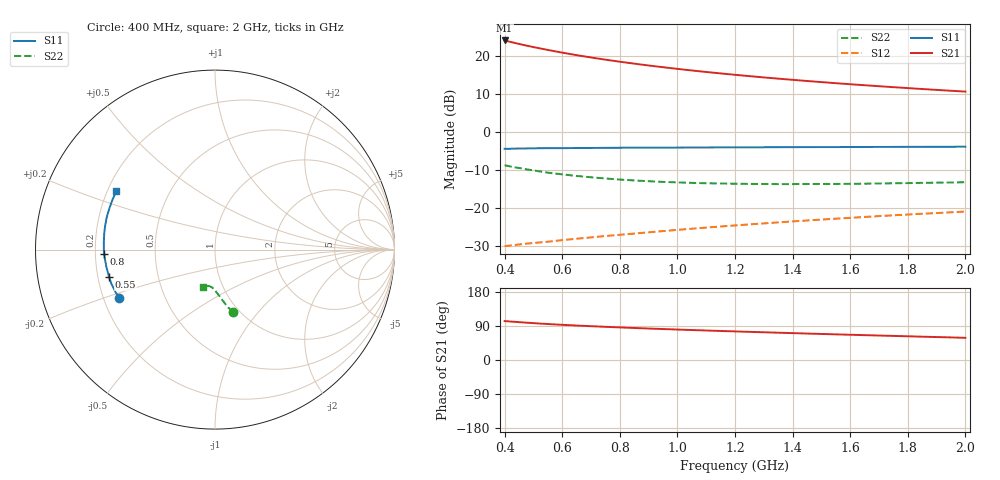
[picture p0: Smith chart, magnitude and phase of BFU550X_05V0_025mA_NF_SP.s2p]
! Filename:  P:\Prog\Test\Noise\ATS_data\Testdata_Net\BFU550X attenuator noise\BFU550X_APG2013_44_C05_05p0V_025mA_NF_CM01_D.sf
! Date/Time: Fri 26/Jul/2013 14:34:21
! BFU550X_APG2013_44_C05_05p0V_1to35mA_NF_CM01_Bias7_R.sf
! Noise Parameter Data File
! BFU550X_APG2013_44_C05_05p0V_1to35mA_NF_CM01
! Date/time: Mon Jul 22 09:12:23 2013
! VAR V_out= 5.001000
! VAR I_out= 25.005000
! VAR V_in= 0.825600
! VAR I_in= 0.279550
! Device data file deembeded for feedlines and parallel
! Original file: \BFU550X attenuator noise\BFU550X_APG2013_44_C05_05p0V_025mA_NF_CM01_R.sf
! Feed-files: PR005V01_100713_Feed1.s2p, PR005V01_100713_Feed2.s2p
! Parallel-file: PR005V01_100713_Par.s2p
# MHz S MA R 50
!  Freq-MHz  S11-mag  S11-arg  S21-mag  S21-arg  S12-mag  S12-arg  S22-mag  S22-arg
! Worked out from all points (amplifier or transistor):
!   37 points, 400 MHz to 2 GHz, reference 50 ohm
!   highest |S21| = 24.0 dB at 400 MHz (marker M1)
!   |S21| within 3 dB of that: start of sweep to 586.2 MHz
!   unconditionally stable (mu >= 1): 1.335 GHz to end of sweep
!   at 500 MHz: K = 0.69, MSG = 25.7 dB, |S12| = -29.2 dB
!   at 1.1 GHz: K = 0.96, MSG = 20.4 dB, |S12| = -25.1 dB
!   at 2 GHz: K = 1.05, MAG = 14.4 dB, |S12| = -20.9 dB
!   lowest NFmin = 1.11 dB at 480 MHz
!   S11 on the Smith chart (normalised r, x): 400 MHz: 0.26, -0.22; 550 MHz: 0.25, -0.12; 800 MHz: 0.24, -0.02; 2 GHz: 0.24, +0.26
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400  0.5995 -153.4  15.81 102.8  0.03158 47.9  0.3643 -74.0
420  0.5995 -155.2  15.13 101.6  0.03225 48.2  0.3512 -75.3
460  0.6038 -158.6  13.96 99.3  0.03356 48.5  0.3314 -77.2
480  0.6057 -160.2  13.43 98.3  0.03418 48.8  0.3198 -78.2
500  0.6076 -161.7  12.95 97.3  0.03476 49.0  0.312 -78.9
550  0.6103 -165.3  11.87 94.9  0.03612 49.9  0.2911 -80.9
600  0.6102 -168.1  10.95 92.9  0.0379 50.7  0.2767 -82.6
650  0.613 -170.8  10.14 91.0  0.03954 51.4  0.2635 -84.1
700  0.6138 -173.2  9.455 89.2  0.04115 52.2  0.253 -85.6
750  0.6161 -175.5  8.849 87.6  0.04293 52.9  0.2441 -86.9
800  0.6183 -177.6  8.321 86.0  0.04455 53.5  0.2364 -88.3
850  0.6193 -179.7  7.848 84.5  0.04621 54.1  0.23 -89.5
900  0.6194 178.5  7.421 83.1  0.04799 54.8  0.2248 -90.6
950  0.6207 176.7  7.045 81.7  0.04981 55.3  0.2202 -91.6
1050  0.622 173.4  6.387 79.1  0.05352 56.2  0.2137 -93.6
1100  0.6235 171.9  6.101 77.8  0.05536 56.6  0.2113 -94.5
1200  0.6253 168.9  5.602 75.4  0.05908 57.2  0.2083 -96.3
1350  0.6283 164.8  4.987 72.0  0.0648 57.9  0.206 -98.8
1500  0.6306 160.9  4.493 68.8  0.07053 58.1  0.2068 -101.2
1600  0.632 158.4  4.213 66.6  0.07434 58.3  0.2077 -102.6
1750  0.634 154.9  3.854 63.6  0.08023 58.3  0.2111 -104.9
2000  0.6383 149.5  3.371 58.6  0.08984 58.0  0.218 -108.4
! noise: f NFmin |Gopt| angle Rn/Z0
400  1.175  0.3291  -172.2  0.0741
460  1.13  0.3594  -172.5  0.0642
600  1.139  0.3797  -168.9  0.0616
800  1.159  0.402  -169.5  0.0566
1000  1.167  0.4102  -164.8  0.0595
1200  1.216  0.4253  -163.7  0.0591
1400  1.26  0.4196  -157.4  0.0694
1600  1.259  0.4999  -154.9  0.0557
1800  1.265  0.4441  -153.6  0.0739
2000  1.315  0.4411  -149.5  0.0889
